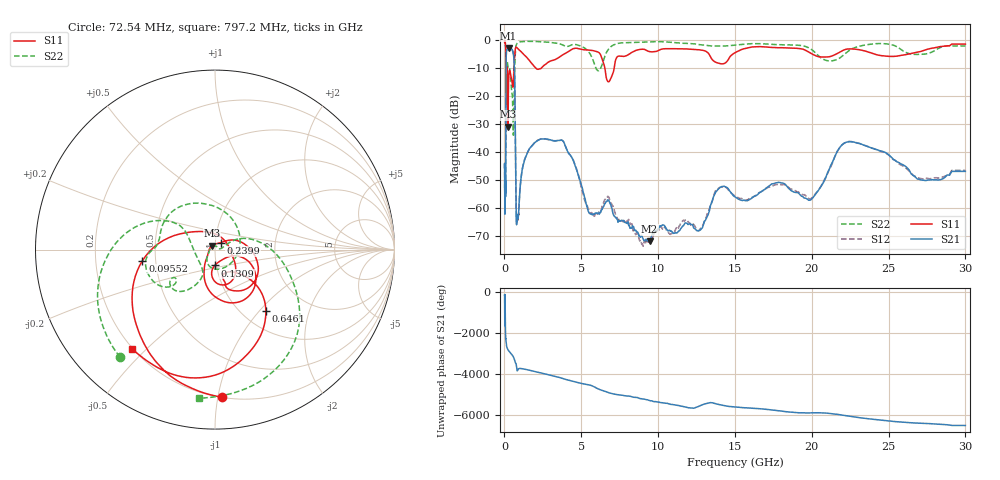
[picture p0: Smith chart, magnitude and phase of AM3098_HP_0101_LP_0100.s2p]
! Date/Time: Thu, Feb 28, 2019 8:36 AM
! Network Analyzer: Agilent Technologies E8364B Rev: A.07.50.67
! Sweep from 0.010 to 30.000 GHz, 1601 Points, Sweep Type: LOG
! Power Supply: 5.022 V, 0.002 A
# Hz S DB R 50
!freq MagS11 AngS11 MagS21 AngS21 MagS12 AngS12 MagS22 AngS22
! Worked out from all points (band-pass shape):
!   1601 points, 10 MHz to 30 GHz, reference 50 ohm
!   highest |S21| = -3.05 dB at 266.5 MHz (marker M1); lowest = -71.9 dB at 9.443 GHz (marker M2)
!   |S21| within 3 dB of the highest: 113.3 MHz to 601.9 MHz (488.6 MHz wide, 137 % of centre)
!   lowest |S11| = -31.1 dB at 230.5 MHz (marker M3), VSWR 1.06, Z = 48.4 + j2.19 ohm
!   |S11| at or under -10 dB: 176.9 MHz to 619.2 MHz (442.3 MHz wide, 111 % of centre); 2.012 GHz to 2.426 GHz (414.2 MHz wide, 18.7 % of centre); 6.528 GHz to 7.146 GHz (618.4 MHz wide, 9.05 % of centre)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
!   |S22| runs from -34.1 to -0.5 dB; largest |S21 - S12| = 0.011
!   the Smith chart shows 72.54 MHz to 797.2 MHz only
!   S11 on the Smith chart (normalised r, x): 72.54 MHz: 0.20, -1.03; 95.52 MHz: 0.42, -0.06; 130.9 MHz: 0.98, -0.17; 239.9 MHz: 1.06, +0.08; 646.1 MHz: 1.28, -1.08; 797.2 MHz: 0.20, -0.45
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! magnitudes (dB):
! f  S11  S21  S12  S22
! 10 MHz  -0.3  -45.8  -44.2  -0.5
! 38.04 MHz  -0.5  -58.5  -60.2  -0.8
! 72.54 MHz  -1.7  -53.0  -52.8  -1.9
! 82.62 MHz  -2.7  -47.1  -47.1  -2.9
! 95.52 MHz  -7.8  -21.5  -21.4  -9.3
! 130.9 MHz  -21.1  -4.4  -4.3  -10.8
! 144.7 MHz  -16.8  -3.8  -3.7  -10.8
! 184.9 MHz  -10.8  -3.6  -3.5  -8.0
! 230.5 MHz  -31.1  -3.1  -3.1  -9.6
! 239.9 MHz  -26.2  -3.1  -3.1  -9.8
! 266.5 MHz  -15.2  -3.0  -3.0  -10.0
! 550.5 MHz  -16.9  -4.4  -4.3  -30.0
! 646.1 MHz  -7.1  -10.2  -10.2  -15.3
! 797.2 MHz  -2.8  -64.5  -64.9  -1.6
! 2.084 GHz  -10.4  -36.3  -36.2  -0.7
! 3.798 GHz  -5.4  -36.1  -36.1  -2.0
! 5.584 GHz  -3.8  -62.1  -62.0  -5.2
! 7.926 GHz  -5.8  -65.3  -65.0  -1.1
! 9.443 GHz  -4.3  -71.9  -71.7  -0.9
! 19.9 GHz  -4.8  -57.3  -56.9  -3.3
! 22.67 GHz  -3.4  -36.5  -36.5  -3.2
! 30 GHz  -1.6  -47.0  -46.6  -2.3
